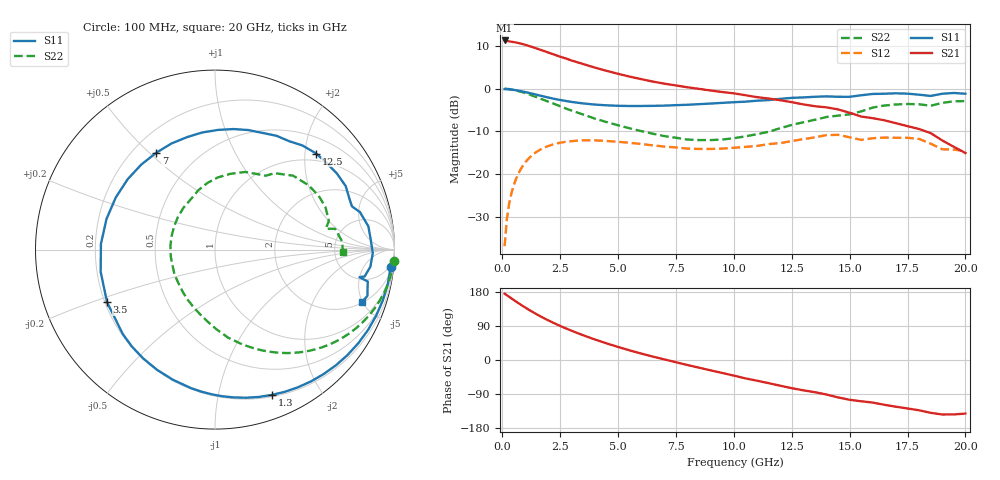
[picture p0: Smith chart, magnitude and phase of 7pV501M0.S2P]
! Infineon Technologies  Discrete & RF Semiconductors
! bfp620
! VCE = 0.50 V,  IC =  1.0 mA
! Common Emitter S-Parameters:  Sep 2002
# GHz  S  MA  R  50
!  f  S11  S21  S12  S22
! GHz  MAG  ANG  MAG  ANG  MAG  ANG  MAG  ANG
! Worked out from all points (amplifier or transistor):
!   59 points, 100 MHz to 20 GHz, reference 50 ohm
!   highest |S21| = 11.3 dB at 100 MHz (marker M1)
!   |S21| within 3 dB of that: start of sweep to 2.078 GHz
!   unconditionally stable (mu >= 1): 6.373 GHz to 15.81 GHz; 17.34 GHz to end of sweep
!   at 1 GHz: K = 0.14, MSG = 13.7 dB, |S12| = -17.2 dB
!   at 5.5 GHz: K = 0.84, MSG = 7.7 dB, |S12| = -12.7 dB
!   at 20 GHz: K = 2.19, MAG = -6.4 dB, |S12| = -14.7 dB
!   S11 on the Smith chart (normalised r, x): 100 MHz: 3, -20; 1.3 GHz: 0.22, -1.44; 3.5 GHz: 0.21, -0.22; 7 GHz: 0.29, +0.53; 12.5 GHz: 0.83, +2.25; 20 GHz: 2.06, -4.93
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0.1  0.9842 -5.6  3.653 175.1  0.0143 85.7  0.9998 -3.6
0.2  0.9815 -11.2  3.603 170.9  0.0301 82.5  0.9932 -7.2
0.5  0.9629 -27.8  3.492 158.1  0.0747 72.2  0.9614 -17.1
0.9  0.9207 -48.8  3.302 142.0  0.1261 58.3  0.9 -29.1
1.3  0.8696 -68.6  3.058 127.1  0.1669 45.9  0.8269 -39.8
1.8  0.8064 -91.3  2.749 110.3  0.2027 32.5  0.7347 -51.3
2.4  0.7433 -115.8  2.41 92.6  0.2293 19.2  0.6364 -63.0
3  0.6964 -137.6  2.125 77.0  0.2426 7.7  0.5515 -73.7
3.5  0.6691 -154.0  1.932 65.1  0.2483 -0.6  0.4956 -81.6
4  0.6489 -169.0  1.758 54.1  0.2475 -8.1  0.445 -88.8
5  0.6281 164.2  1.487 34.4  0.2382 -19.5  0.3715 -102.6
6  0.6249 141.2  1.288 17.0  0.2242 -28.3  0.3178 -118.7
7  0.6309 121.3  1.14 1.6  0.2093 -33.9  0.2776 -136.7
8.5  0.6565 96.2  0.991 -20.3  0.1964 -37.9  0.2495 -170.9
10.5  0.7023 67.7  0.835 -48.6  0.2076 -42.1  0.2756 138.4
12.5  0.7776 43.5  0.693 -74.4  0.2428 -50.2  0.3749 96.2
13.5  0.8008 31.9  0.621 -85.0  0.2686 -58.0  0.4308 78.5
15  0.8002 17.5  0.521 -105.0  0.2688 -79.5  0.4989 55.6
16  0.8644 8.6  0.45 -112.4  0.2621 -81.8  0.5992 43.4
17  0.8792 -1.3  0.393 -123.3  0.2653 -93.1  0.651 27.4
18.5  0.8193 -10.8  0.301 -139.4  0.2265 -115.0  0.6283 10.7
20  0.8691 -19.7  0.176 -141.4  0.1845 -118.3  0.7131 -0.9
